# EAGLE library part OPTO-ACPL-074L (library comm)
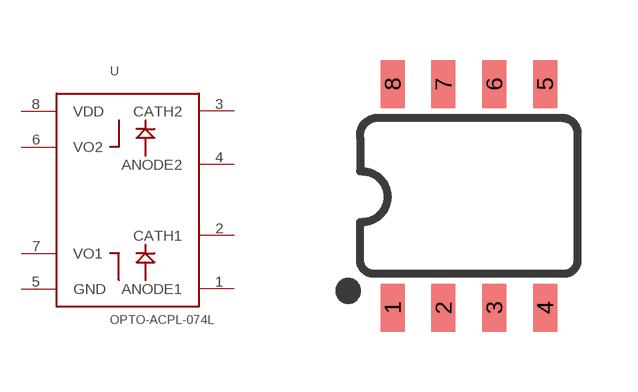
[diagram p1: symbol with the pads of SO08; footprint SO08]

Designator prefix U

## OPTO-ACPL-074LSOIC  [SO08]
1  ANODE1
2  CATH1
3  CATH2
4  ANODE2
5  GND
6  VO2
7  VO1
8  VDD

## Footprint SO08 (pad centres in mm)
SOIC, 0.15 inch width
smd 0.6 x 1.2: 1 -1.905,-2.8; 2 -0.635,-2.8; 3 0.635,-2.8; 4 1.905,-2.8; 5 1.905,2.8; 6 0.635,2.8; 7 -0.635,2.8; 8 -1.905,2.8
